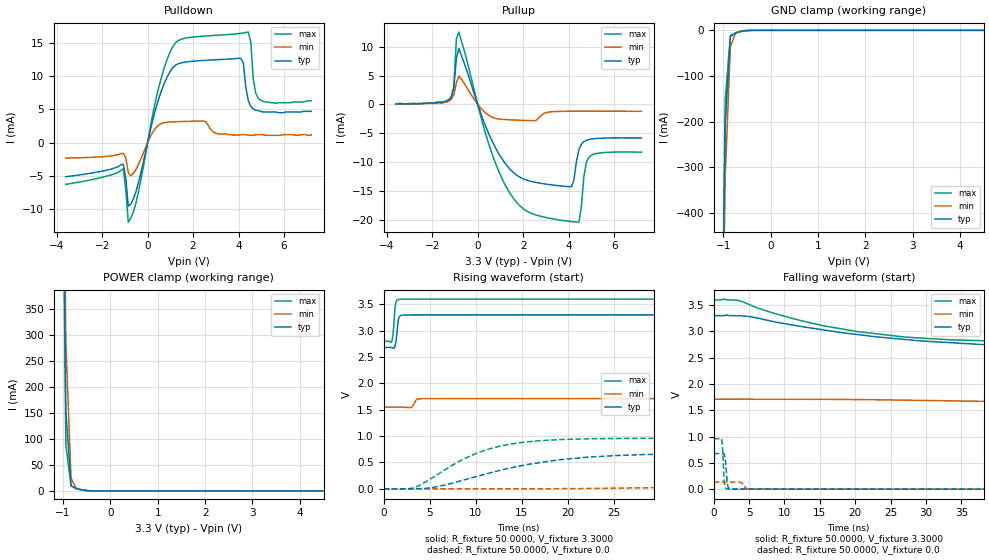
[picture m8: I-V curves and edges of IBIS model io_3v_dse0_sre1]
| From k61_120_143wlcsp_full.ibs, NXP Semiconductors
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[Model]  io_3v_dse0_sre1
|   Model io_3v_dse0_sre1
| Library cells for typ/min/max conditions are connected as defined below:
|  pad - External Pad
|  ipp_do_3v - Core Input
|  ipp_obe_3v - Output Buffer Enable
|  esd_boost - vdd_s_3v
|  esd_trigger - vss_s_3v
|  ipp_ame_3v - vss_s_3v
|  ipp_dse_3v - vss_s_3v
|  ipp_ina_3v - NC
|  ipp_ina_mux_3v - NC
|  ipp_ind_3v - NC
|  ipp_pue_3v - vss_s_3v
|  ipp_sre_3v - vdd_s_3v
|  tie_3v - vdd_s_3v
|  tie_hi - vdd_s_lv
|  vbuf_3v - vdd_s_3v
|  vdd_s_3v - vdd_s_3v
|  vdd_s_lv - vdd_s_lv
|  vss_bulk - vss_s_3v
|  vss_s_3v - vss_s_3v
| All other pins connected to ground
Model_type I/O
Polarity   Non-Inverting
Enable   Active-High
Vinl =   1.1550V
Vinh =   2.3100V
Vmeas =  1.6500V
Cref =   25.0000pF
Rref =   50.0000
Vref =   0.0V
C_comp   1.9040pF   1.7928pF   2.1191pF
[Temperature Range]   25.0000   0.1250k   -40.0000
[Voltage Range]   3.3000V   1.7100V   3.6000V
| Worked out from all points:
|   slope of the pulldown table from 0 to 0.495 V, typ, clamps not added: 74.6 ohm
|   slope of the pullup table from 0 to 0.495 V, typ, clamps not added: 96.1 ohm
|   GND clamp passes 1 mA (typ) near -0.54 V on its own axis
|   POWER clamp passes 1 mA (typ) near -0.53 V on its own axis
|   rising waveform, R_fixture 50.0000, V_fixture 3.3000: 20-80 % time 232ps typ, 307ps min, 203ps max; typ from 2.68 V to 3.3 V
|   rising waveform, R_fixture 50.0000, V_fixture 0.0: 20-80 % time 10.6ns typ, 34.1ns min, 6.58ns max; typ from 0 V to 0.676 V
|   falling waveform, R_fixture 50.0000, V_fixture 3.3000: 20-80 % time 22.3ns typ, 52ns min, 16.6ns max; typ from 3.3 V to 2.68 V
|   falling waveform, R_fixture 50.0000, V_fixture 0.0: 20-80 % time 254ps typ, 467ps min, 212ps max; typ from 0.676 V to 0 V
[Pulldown]
|Voltage   I(typ)   I(min)   I(max)
-3.6V     -5.11mA    -2.33mA    -6.26mA
-1.07V    -3.221mA   -1.617mA   -3.914mA
-850mV    -9.536mA   -4.465mA   -11.95mA
-520mV    -7.435mA   -4.073mA   -9.159mA
580mV     7.513mA    2.843mA    9.475mA
1.46V     11.97mA    3.168mA    15.51mA
4.1V      12.68mA    1.2mA      16.42mA
4.43V     6.32mA     1.1mA      16.6mA
4.54V     5.46mA     1.1mA      15.13mA
4.65V     5.07mA     1.1mA      9.53mA
4.87V     4.8mA      1.2mA      6.66mA
7.2V      4.7mA      1.2mA      6.3mA
[Pullup]
|Voltage   I(typ)   I(min)   I(max)
-3.6V     100uA      0A         100uA
-1.27V    830uA      570uA      820uA
-1.05V    2.86mA     1.69mA     3.17mA
-940mV    8.013mA    3.698mA    11.33mA
-830mV    9.687mA    4.912mA    12.52mA
710mV     -6.946mA   -2.313mA   -9.402mA
2.14V     -13.06mA   -2.762mA   -18.39mA
4.12V     -14.22mA   -1.16mA    -20.25mA
4.45V     -7.839mA   -1.16mA    -20.35mA
4.67V     -6.422mA   -1.16mA    -12.47mA
4.89V     -6.059mA   -1.16mA    -9.139mA
7.2V      -5.79mA    -1.18mA    -8.25mA
[GND_clamp]
|Voltage   I(typ)   I(min)   I(max)
-3.6V     -47.78A    -47.06A    -48.3A
-1.07V    -1.101A    -1.183A    -1.105A
-960mV    -210.7mA   -326mA     -154mA
-850mV    -14.47mA   -36.11mA   -11.11mA
-740mV    -5.262mA   -6.034mA   -5.843mA
-520mV    -637uA     -915.4uA   -467.5uA
-300mV    -2.578uA   -18.09uA   -370.9nA
7.2V      0A         0A         0A
[POWER_clamp]
|Voltage   I(typ)   I(min)   I(max)
-3.6V     52.51A     51.88A     52.98A
-1.05V    1.126A     1.265A     1.065A
-940mV    154.2mA    286.1mA    88.03mA
-830mV    9.989mA    24.5mA     9.181mA
-720mV    4.227mA    4.408mA    5.116mA
-390mV    66.57uA    164uA      29.9uA
7.2V      0A         0A         0A
[Ramp]
| variable   typ   min   max
dV/dt_r  0.4058/10.6214n   80.3142m/34.1271n   0.5757/6.5774n
dV/dt_f  0.3717/22.2614n   95.2506m/51.9799n   0.4823/16.5966n
R_load = 50.0000
[Rising Waveform]
R_fixture= 50.0000
V_fixture= 3.3000
V_fixture_min= 1.7100
V_fixture_max= 3.6000
|time   V(typ)   V(min)   V(max)
0s        2.681V     1.551V     2.796V
861.3ps   2.68V      1.551V     2.789V
1.013ns   2.667V     1.552V     2.924V
1.146ns   2.673V     1.552V     3.221V
1.341ns   2.809V     1.552V     3.542V
1.597ns   3.205V     1.552V     3.593V
1.926ns   3.294V     1.552V     3.598V
2.988ns   3.299V     1.545V     3.599V
4.271ns   3.299V     1.71V      3.599V
250ns     3.3V       1.71V      3.6V
[Rising Waveform]
R_fixture= 50.0000
V_fixture= 0.0
V_fixture_min= 0.0
V_fixture_max= 0.0
|time   V(typ)   V(min)   V(max)
0s        5.331nV    455.6nV    4.026nV
3.341ns   -72.51uV   -1.47mV    23.77mV
5.094ns   19mV       -43.96uV   188.3mV
8.601ns   161.6mV    -18.39uV   560mV
12.62ns   348.9mV    95.22uV    809.2mV
17.02ns   498.4mV    1.343mV    913.8mV
22.1ns    599.9mV    6.091mV    948.6mV
35.46ns   668.9mV    36.95mV    959.2mV
84.61ns   676.3mV    125mV      959.6mV
250ns     676.3mV    133.9mV    959.6mV
[Falling Waveform]
R_fixture= 50.0000
V_fixture= 3.3000
V_fixture_min= 1.7100
V_fixture_max= 3.6000
|time   V(typ)   V(min)   V(max)
0s        3.3V       1.71V      3.6V
3.517ns   3.3V       1.71V      3.589V
7.042ns   3.228V     1.71V      3.408V
12.25ns   3.097V     1.71V      3.208V
20.29ns   2.942V     1.705V     2.998V
27.15ns   2.846V     1.693V     2.892V
39.62ns   2.741V     1.667V     2.818V
57.25ns   2.693V     1.629V     2.799V
112.5ns   2.681V     1.564V     2.796V
250ns     2.681V     1.551V     2.796V
[Falling Waveform]
R_fixture= 50.0000
V_fixture= 0.0
V_fixture_min= 0.0
V_fixture_max= 0.0
|time   V(typ)   V(min)   V(max)
0s        676.3mV    133.9mV    959.6mV
1.108ns   677.7mV    133.8mV    943.8mV
1.236ns   680mV      133.8mV    800.9mV
1.524ns   643.9mV    133.7mV    102.4mV
1.654ns   537.1mV    133.7mV    29.51mV
1.934ns   99.66mV    133.7mV    3.715mV
2.129ns   17.36mV    133.7mV    2.081mV
3.819ns   689.8uV    129.1mV    845.9uV
5.381ns   494.6uV    281.1uV    592uV
250ns     13.63nV    207nV      11.46nV
